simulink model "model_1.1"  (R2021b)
settings: Solver=VariableStepAuto  StartTime=0.0  StopTime=20  RelTol=1e-3
undefined symbols (not defined in the file or in its folder): dynamics
libraries: fl_lib x17, nesl_utility x7, sdl_lib x1

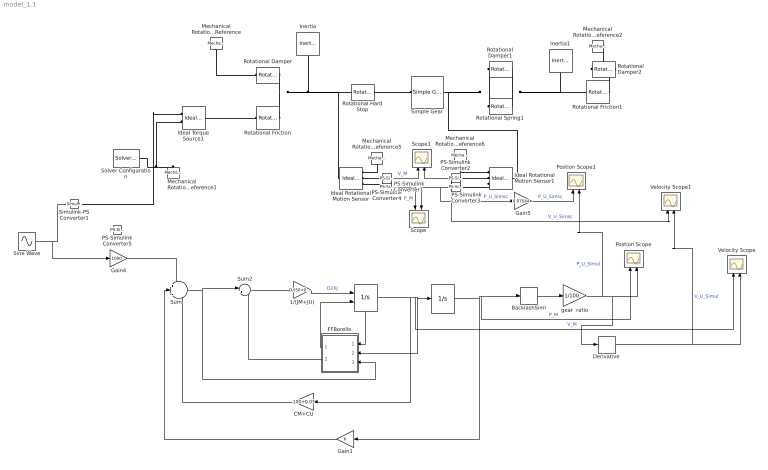
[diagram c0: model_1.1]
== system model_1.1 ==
  " " : Integrator  ExternalReset=rising  ShowStatePort=on
  "  " : Integrator  UpperSaturationLimit=dynamics.ThUmax/dynamics.tau  LowerSaturationLimit=dynamics.ThUmin/dynamics.tau
  1/(JM+JU) : Gain  Gain=1/(50+0.085)%1/(dynamics.JM+dynamics.JU)
  BacklashSiml : Backlash  BacklashWidth=0.0035
  CM+CU : Gain  Gain=100+0.03
  Derivative : Derivative
  FFBorello : Subsystem
  Gain1 : Gain
  Gain4 : Gain  Gain=1000
  Gain5 : Gain  Gain=0.07544
  Ideal Rotational Motion Sensor : fl_lib/Mechanical/Mechanical Sensors/Ideal Rotational Motion Sensor  wrap_angle=simscape.enum.onoff.off  offset=0 rad
  Ideal Rotational Motion Sensor1 : fl_lib/Mechanical/Mechanical Sensors/Ideal Rotational Motion Sensor  wrap_angle=simscape.enum.onoff.off  offset=0 rad
  Ideal Torque Source1 : fl_lib/Mechanical/Mechanical Sources/Ideal Torque Source
  Inertia : fl_lib/Mechanical/Rotational Elements/Inertia  inertia=0.085 kg*m^2  num_ports=foundation.enum.numPorts2.one  w_specify=off  w_priority=High  w=0 rad/s  w_nominal_specify=off  w_nominal_unit=rad/s  w_nominal_value=1  t_specify=off  t_priority=None  t=0 N*m  t_nominal_specify=off  t_nominal_unit=N*m  t_nominal_value=1
  Inertia1 : fl_lib/Mechanical/Rotational Elements/Inertia  inertia=50 kg*m^2  num_ports=foundation.enum.numPorts2.one  w_specify=off  w_priority=High  w=0 rad/s  w_nominal_specify=off  w_nominal_unit=rad/s  w_nominal_value=1  t_specify=off  t_priority=None  t=0 N*m  t_nominal_specify=off  t_nominal_unit=N*m  t_nominal_value=1
  Mechanical Rotational Reference{,1..2,5..6} (5 alike) : fl_lib/Mechanical/Rotational Elements/Mechanical Rotational Reference
  PS-Simulink Converter{1..5} (5 alike) : nesl_utility/PS-Simulink Converter  PhysicalDomain=network_engine_domain  SubClassName=ps_output  LeftPortType=input  RightPortType=output  PseudoPeriodic=off  Frequencies=[]  Unit=inherit  AffineConversion=off
  Postion Scope : Scope  NumInputPorts=2
  Postion Scope1 : Scope  NumInputPorts=2
  Rotational Damper : fl_lib/Mechanical/Rotational Elements/Rotational Damper  D=0.03 N*m/(rad/s)  w_specify=off  w_priority=None  w=0 rad/s  w_nominal_specify=off  w_nominal_unit=rad/s  w_nominal_value=1  t_specify=off  t_priority=None  t=0 N*m  t_nominal_specify=off  t_nominal_unit=N*m  t_nominal_value=1
  Rotational Damper1 : fl_lib/Mechanical/Rotational Elements/Rotational Damper  D=5e1 N*m/(rad/s)  w_specify=off  w_priority=None  w=0 rad/s  w_nominal_specify=off  w_nominal_unit=rad/s  w_nominal_value=1  t_specify=off  t_priority=None  t=0 N*m  t_nominal_specify=off  t_nominal_unit=N*m  t_nominal_value=1
  Rotational Damper2 : fl_lib/Mechanical/Rotational Elements/Rotational Damper  D=100 N*m/(rad/s)  w_specify=off  w_priority=None  w=0 rad/s  w_nominal_specify=off  w_nominal_unit=rad/s  w_nominal_value=1  t_specify=off  t_priority=None  t=0 N*m  t_nominal_specify=off  t_nominal_unit=N*m  t_nominal_value=1
  Rotational Friction : fl_lib/Mechanical/Rotational Elements/Rotational Friction  brkwy_trq=5 N*m  brkwy_vel=0.1 rad/s  Col_trq=5 N*m  visc_coef=0 N*m/(rad/s)  w_specify=off  w_priority=None  w=0 rad/s  w_nominal_specify=off  w_nominal_unit=rad/s  w_nominal_value=1  t_specify=off  t_priority=None  t=0 N*m  t_nominal_specify=off  t_nominal_unit=N*m  t_nominal_value=1
  Rotational Friction1 : fl_lib/Mechanical/Rotational Elements/Rotational Friction  brkwy_trq=500 N*m  brkwy_vel=0.1 rad/s  Col_trq=500 N*m  visc_coef=0 N*m/(rad/s)  w_specify=off  w_priority=None  w=0 rad/s  w_nominal_specify=off  w_nominal_unit=rad/s  w_nominal_value=1  t_specify=off  t_priority=None  t=0 N*m  t_nominal_specify=off  t_nominal_unit=N*m  t_nominal_value=1
  Rotational Hard Stop : fl_lib/Mechanical/Rotational Elements/Rotational Hard Stop  upper_bnd=1 deg  lower_bnd=-1 deg  stiff_up=1e6 N*m/rad  stiff_low=1e6 N*m/rad  D_up=0.01 N*m/(rad/s)  D_low=0.01 N*m/(rad/s)  model=simscape.enum.hardstop.smooth  transition=0.001 rad  w_specify=off  w_priority=None  w=0 rad/s  w_nominal_specify=off  w_nominal_unit=rad/s  w_nominal_value=1  t_specify=off  t_priority=None  t=0 N*m  t_nominal_specify=off  t_nominal_unit=N*m  t_nominal_value=1  phi_specify=off  phi_priority=High  phi=0 rad  phi_nominal_specify=off  phi_nominal_unit=rad  phi_nominal_value=1
  Rotational Spring1 : fl_lib/Mechanical/Rotational Elements/Rotational Spring  spr_rate=5e1 N*m/rad  w_specify=off  w_priority=None  w=0 rad/s  w_nominal_specify=off  w_nominal_unit=rad/s  w_nominal_value=1  t_specify=off  t_priority=None  t=0 N*m  t_nominal_specify=off  t_nominal_unit=N*m  t_nominal_value=1  phi_specify=off  phi_priority=High  phi=0 rad  phi_nominal_specify=off  phi_nominal_unit=rad  phi_nominal_value=1
  Scope : Scope  NumInputPorts=2
  Scope1 : Scope  NumInputPorts=2
  Simple Gear : sdl_lib/Gears/Simple Gear  ratio=100  rotation_direction=sdl.enum.shaftOutputDirection.same  friction_model=sdl.enum.gear_efficiencies_load.off  T_noload=0.1 N*m  T_nom=5 N*m  efficiency_nom=0.8  efficiency=0.8  temperature_TLU=[280, 300, 320] K  load_TLU=[1, 5, 10] N*m  efficiency_TLU=[.95, .9, .85]  efficiency_TLU2=[.85, .8, .75; .95, .9, .85; .85, .8, .7]  w_thr=0.01 rad/s  pwr_thr=0.001 W  backlash_model=sdl.enum.backlashModel.Off  backlash_distance=1e-3 mm  x0=0 mm  r_base=0.1 m  hardstop_model=simscape.enum.hardstop.smooth  transition=1e-4 mm  backlash_stiffness=1e7 N/m  backlash_damping=1e6 N/(m/s)  e=0  v_tol=0.001 m/s  mu_visc=[0, 0] N*m/(rad/s)  enable_faults=simscape.enum.onoff.off  efficiency_fault=0.05  external_fault=simscape.enum.onoff.off  temporal_fault=simscape.enum.onoff.off  fault_time=5 s  fault_angles=pi / 12 rad  report_fault=simscape.enum.assert.action.none  thermal_mass=50 J/K  temperature_specify=off  temperature_priority=High  temperature=300 K  temperature_nominal_specify=off  temperature_nominal_unit=K  temperature_nominal_value=1
  Simulink-PS Converter1 : nesl_utility/Simulink-PS Converter  PhysicalDomain=network_engine_domain  SubClassName=ps_input  LeftPortType=input  RightPortType=output  PseudoPeriodic=off  Frequencies=[]  NoiseDistribution=none  NoiseParameters=[]  Unit=1  AffineConversion=off  FilteringAndDerivatives=provide  SimscapeFilterOrder=1  InputFilterTimeConstant=0.001  UdotUserProvided=0
  Sine Wave : Sin  Frequency=10  SampleTime=0
  Solver Configuration : nesl_utility/Solver Configuration  PhysicalDomain=network_engine_domain  SubClassName=solver  LeftPortType=input  RightPortType=generic  Tones=[]  Harmonics=[]  SimulateNoise=off  Profile=off  UseLocalSampling=off  EnableSwitchedLinearOptims=on  FrequencyDomain=off  UseCCode=off  RelTol=0.001  AbsTol=1e-06  MinStep=1e-09  ToWorkspace=off  RevertToSquareIcSolve=off  NumHomotopyIterations=100  PhasorMode=off  PhasorModeNumHarmonics=1  DoDC=off  ResidualTolerance=1e-09  UseLocalSolver=off  LocalSolverChoice=NE_BACKWARD_EULER_ADVANCER  LocalSolverSampleTime=0.001  DoFixedCost=off  MaxNonlinIter=3  MaxModeIter=2  ComputeImpulses=off  ImpulseIterations=2  LinearAlgebra=auto  EquationFormulation=NE_TIME_EF  DelaysMemoryBudget=1024  AutomaticFiltering=on  FilteringTimeConstant=0.001  PartitionStorageMethod=AS_NEEDED  PartitionMemoryBudget=1024  PartitionMethod=ROBUST
  Sum : Sum  Inputs=+--
  Sum2 : Sum  Inputs=|+-
  Velocity Scope : Scope  NumInputPorts=2
  Velocity Scope1 : Scope  NumInputPorts=2
  gear  ratio : Gain  Gain=1/100
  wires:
  PS-Simulink Converter2/1 -> Velocity Scope1/1, Scope1/2  "V_U_Simsc"
  PS-Simulink Converter4/1 -> Scope1/1  "V_M"
  PS-Simulink Converter1/1 -> Scope/1  "P_M"
  " "/State -> FFBorello/1(DXJ SP)
  gear  ratio/1 -> Postion Scope/2, Derivative/1, Postion Scope1/2  "P_U_Simul"
  Derivative/1 -> Velocity Scope/2, Velocity Scope1/2  "V_U_Simul"
  BacklashSiml/1 -> gear  ratio/1
  " "/1 -> Velocity Scope/1, "  "/1, FFBorello/2(DXJ), CM+CU/1  "V_M"
  1/(JM+JU)/1 -> " "/1  "D2XJ"
  FFBorello/1(Reset_DXJ) -> " "/2
  Sum/1 -> FFBorello/3(Act Torque), Sum2/1
  Gain1/1 -> Sum/2
  CM+CU/1 -> Sum/3
  Sum2/1 -> 1/(JM+JU)/1
  FFBorello/2(TF) -> Sum2/2
  "  "/1 -> Gain1/1, Postion Scope/1, BacklashSiml/1  "P_M"
  PS-Simulink Converter3/1 -> Gain5/1, Scope/2  "P_U_Simsc"
  Sine Wave/1 -> Gain4/1, Simulink-PS Converter1/1
  Gain4/1 -> Sum/1
  Gain5/1 -> Postion Scope1/1  "P_U_Simsc"
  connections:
  Mechanical Rotational Reference/LConn1 -- Rotational Damper/LConn1
  Ideal Torque Source1/LConn1 -- Rotational Friction/LConn1
  Rotational Friction/RConn1 -- Ideal Rotational Motion Sensor/LConn1 -- Rotational Hard Stop/LConn1 -- Inertia/LConn1 -- Rotational Damper/RConn1
  Mechanical Rotational Reference1/LConn1 -- Solver Configuration/RConn1 -- Ideal Torque Source1/RConn2
  Rotational Hard Stop/RConn1 -- Simple Gear/LConn1
  Rotational Damper1/LConn1 -- Ideal Rotational Motion Sensor1/LConn1 -- Simple Gear/RConn1 -- Rotational Spring1/LConn1
  Rotational Damper1/RConn1 -- Inertia1/LConn1 -- Rotational Friction1/LConn1 -- Rotational Spring1/RConn1
  Rotational Damper2/RConn1 -- Rotational Friction1/RConn1
  Ideal Rotational Motion Sensor1/RConn3 -- PS-Simulink Converter3/LConn1
  PS-Simulink Converter2/LConn1 -- Ideal Rotational Motion Sensor1/RConn2
  Mechanical Rotational Reference5/LConn1 -- Ideal Rotational Motion Sensor/RConn1
  Mechanical Rotational Reference6/LConn1 -- Ideal Rotational Motion Sensor1/RConn1
  PS-Simulink Converter1/LConn1 -- Ideal Rotational Motion Sensor/RConn3
  PS-Simulink Converter4/LConn1 -- Ideal Rotational Motion Sensor/RConn2
  Mechanical Rotational Reference2/LConn1 -- Rotational Damper2/LConn1
  Simulink-PS Converter1/RConn1 -- Ideal Torque Source1/RConn1

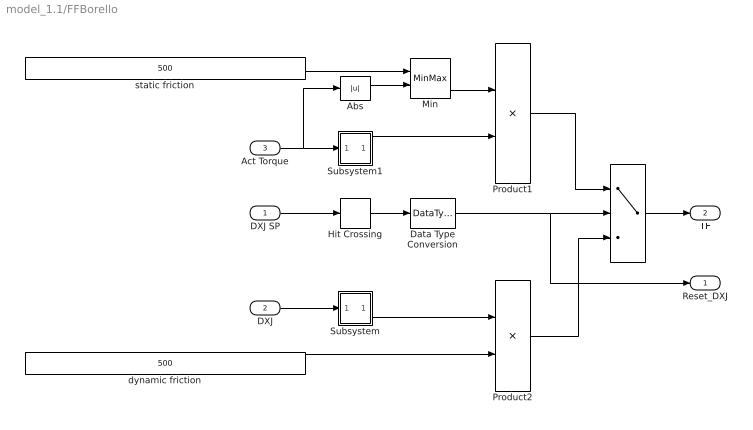
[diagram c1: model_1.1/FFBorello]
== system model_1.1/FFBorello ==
  DXJ SP : Inport
  DXJ : Inport  Port=2
  Act Torque : Inport  Port=3
  "   " : Switch  Threshold=0.5
  Abs : Abs
  Data Type Conversion : DataTypeConversion  OutDataTypeStr=double
  Hit Crossing : HitCross
  Min : MinMax  Inputs=2  InputSameDT=on  SaturateOnIntegerOverflow=on
  Product1 : Product  InputSameDT=on  RndMeth=Zero  SaturateOnIntegerOverflow=on
  Product2 : Product  InputSameDT=on  RndMeth=Zero  SaturateOnIntegerOverflow=on
  Subsystem : Subsystem
  Subsystem1 : Subsystem
  dynamic friction : Constant  Value=500
  static friction : Constant  Value=500
  Reset_DXJ : Outport
  TF : Outport  Port=2
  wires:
  Product2/1 -> "   "/3
  DXJ/1 -> Subsystem/1(In1)
  "   "/1 -> TF/1
  Product1/1 -> "   "/1
  Min/1 -> Product1/1
  Act Torque/1 -> Subsystem1/1(In1), Abs/1
  Abs/1 -> Min/2
  Hit Crossing/1 -> Data Type Conversion/1
  Subsystem/1(Out1) -> Product2/1
  Subsystem1/1(Out1) -> Product1/2
  Data Type Conversion/1 -> "   "/2, Reset_DXJ/1
  DXJ SP/1 -> Hit Crossing/1
  static friction/1 -> Min/1
  dynamic friction/1 -> Product2/2

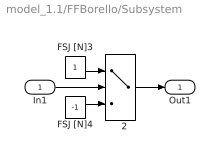
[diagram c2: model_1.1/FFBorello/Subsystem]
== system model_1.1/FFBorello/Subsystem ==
  In1 : Inport
  "   2" : Switch
  FSJ [N]3 : Constant
  FSJ [N]4 : Constant  Value=-1
  Out1 : Outport
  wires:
  FSJ [N]3/1 -> "   2"/1
  FSJ [N]4/1 -> "   2"/3
  In1/1 -> "   2"/2
  "   2"/1 -> Out1/1

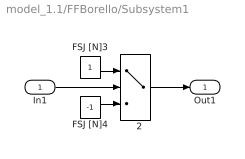
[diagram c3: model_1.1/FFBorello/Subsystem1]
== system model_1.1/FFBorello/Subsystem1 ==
  In1 : Inport
  "   2" : Switch
  FSJ [N]3 : Constant
  FSJ [N]4 : Constant  Value=-1
  Out1 : Outport
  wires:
  FSJ [N]3/1 -> "   2"/1
  FSJ [N]4/1 -> "   2"/3
  In1/1 -> "   2"/2
  "   2"/1 -> Out1/1
